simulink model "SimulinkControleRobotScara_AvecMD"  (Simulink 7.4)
settings: Solver=ode45  StartTime=0.0  StopTime=T  FixedStep=0.1  MaxStep=0.1  MinStep=0.01  RelTol=0.1  AbsTol=0.01
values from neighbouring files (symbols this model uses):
  theta1 = theta1_last+n*Deltatheta1    [GestionGUI.m]    (also in ModeleGeometriqueDirect.m = Theta(1); ModeleGeometriqueInverse.m = alpha - beta; SimulationRobotSCARA.m = 1.57079632679)
  theta2 = theta2_last+n*Deltatheta2    [GestionGUI.m]    (also in ModeleGeometriqueDirect.m = Theta(2); ModeleGeometriqueInverse.m = acos((x^2+y^2-l1^2-l2^2)/(2*l1*l2)); SimulationRobotSCARA.m = 1.57079632679)
libraries: simulink x3, simulink_extras x2

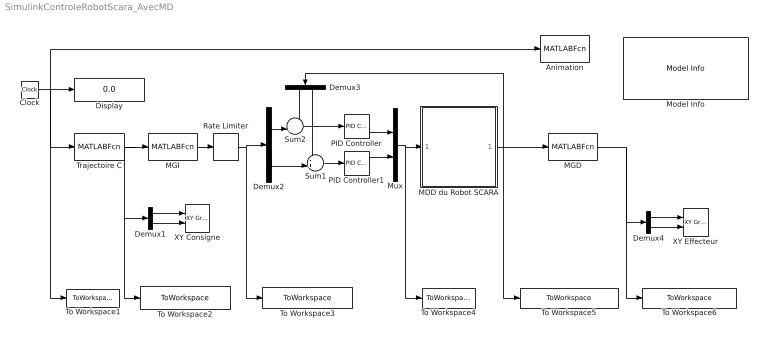
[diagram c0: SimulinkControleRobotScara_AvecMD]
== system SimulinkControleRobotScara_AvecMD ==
  Animation : MATLABFcn  Tag=Affichage  Description=Affichage  MATLABFcn=SetAffichage  OutputDimensions=0
  Clock : Clock
  Demux{1..4} (4 alike) : Demux  Outputs=2
  Display : Display
  MDD du Robot SCARA : Subsystem  Tag=Robot  Description=Robot
  MGD : MATLABFcn  MATLABFcn=ModeleGeometriqueDirect  OutputDimensions=2
  MGI : MATLABFcn  MATLABFcn=ModeleGeometriqueInverse  OutputDimensions=2
  Model Info : simulink/Model-Wide Utilities/Model Info  SystemSampleTime=-1  InitialBlockCM=None  BlockCM=None  Frame=on  DisplayStringWithTags=|  HorizontalTextAlignment=Left  LeftAlignmentValue=0.02  SourceBlockDiagram=SimulinkControleRobotScara_AvecMD  TagMaxNumber=20
      | Asservissement de position 
      |   d'un robot SCARA 2D
      | 
      |   Lounis Adouane
      |   Polytech'Clermont-Ferrand
  Mux : Mux  Inputs=[1 1]
  PID Controller : simulink_extras/Additional Linear/PID Controller  SystemSampleTime=-1  P=10  I=5  D=2
  PID Controller1 : simulink_extras/Additional Linear/PID Controller  SystemSampleTime=-1  P=10  I=5  D=2
  Rate Limiter : RateLimiter  RisingSlewLimit=200  FallingSlewLimit=-200
  Sum1 : Sum  Inputs=-+|  OutDataType=sfix(16)  OutScaling=2^0
  Sum2 : Sum  Inputs=-+|  OutDataType=sfix(16)  OutScaling=2^0
  To Workspace1 : ToWorkspace  VariableName=DS_Temps  SaveFormat=Array
  To Workspace2 : ToWorkspace  VariableName=DS_PositionConsigne  SaveFormat=Array
  To Workspace3 : ToWorkspace  VariableName=DS_ThetaConsigne  SaveFormat=Array
  To Workspace4 : ToWorkspace  VariableName=DS_Gama  SaveFormat=Array
  To Workspace5 : ToWorkspace  VariableName=DS_ThetaArticulations  SaveFormat=Array
  To Workspace6 : ToWorkspace  VariableName=DS_PositionEffecteur  SaveFormat=Array
  Trajectoire C : MATLABFcn  MATLABFcn=TrajectoireConsigne  OutputDimensions=2
  XY Consigne : simulink/Sinks/XY Graph  SystemSampleTime=-1  xmin=-20  xmax=20  ymin=-3  ymax=20  st=-1
  XY Effecteur : simulink/Sinks/XY Graph  SystemSampleTime=-1  xmin=-20  xmax=20  ymin=-3  ymax=20  st=-1
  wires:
  Mux/1 -> MDD du Robot SCARA/1(Gama), To Workspace4/1
  MDD du Robot SCARA/1(q) -> Demux3/1, MGD/1, To Workspace5/1
  PID Controller/1 -> Mux/1
  PID Controller1/1 -> Mux/2
  Sum2/1 -> PID Controller/1
  Sum1/1 -> PID Controller1/1
  Demux3/1 -> Sum2/1
  Demux3/2 -> Sum1/1
  Demux2/1 -> Sum2/2
  Demux2/2 -> Sum1/2
  Clock/1 -> Display/1, To Workspace1/1, Animation/1, Trajectoire C/1
  Trajectoire C/1 -> Demux1/1, To Workspace2/1, MGI/1
  Demux1/1 -> XY Consigne/1
  Demux1/2 -> XY Consigne/2
  Demux4/1 -> XY Effecteur/1
  Demux4/2 -> XY Effecteur/2
  MGD/1 -> To Workspace6/1, Demux4/1
  MGI/1 -> Rate Limiter/1
  Rate Limiter/1 -> To Workspace3/1, Demux2/1

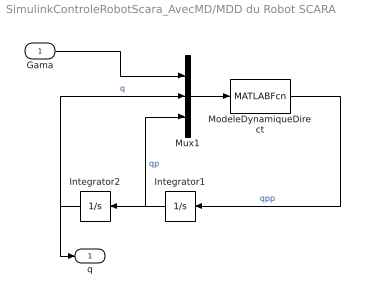
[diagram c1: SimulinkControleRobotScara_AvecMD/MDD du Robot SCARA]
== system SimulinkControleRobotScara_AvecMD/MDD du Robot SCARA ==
  Gama : Inport  OutDataType=sfix(16)  OutScaling=2^0
  Integrator1 : Integrator  InitialCondition=zeros(1,2)
  Integrator2 : Integrator  InitialCondition=[theta1, theta2]
  ModeleDynamiqueDirect : MATLABFcn  MATLABFcn=ModeleDynamiqueDirect  OutputDimensions=2
  Mux1 : Mux  Inputs=[2 2 2]
  q : Outport
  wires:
  Mux1/1 -> ModeleDynamiqueDirect/1
  Integrator1/1 -> Integrator2/1, Mux1/3  "qp"
  ModeleDynamiqueDirect/1 -> Integrator1/1  "qpp"
  Integrator2/1 -> Mux1/2, q/1  "q"
  Gama/1 -> Mux1/1
